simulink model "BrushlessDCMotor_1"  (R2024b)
settings: Solver=ode4  StartTime=0  StopTime=3  FixedStep=Ts  MaxStep=1e-6  RelTol=1e-6  AbsTol=1e-6  EnableMultiTasking=on
PreLoadFcn:
  | assignin('base','Ts',[5e-6])
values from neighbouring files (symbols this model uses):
  A = [-Rs/Ls,  -Ke/Ls    [dc_motor_hinf.m]
  B = 0.001    [dc_motor_hinf.m]
  J = 0.0008    [dc_motor_hinf.m]
  Ke = 0.175    [dc_motor_hinf.m]
  Kt = 0.175    [dc_motor_hinf.m]
  Ls = 8.5e-3    (= 0.0085)    [dc_motor_hinf.m]
  Rs = 2.875    [dc_motor_hinf.m]
  Ts = 5e-6    (= 5e-06)    [dc_motor_hinf.m]
undefined symbols (not defined in the file or in its folder): axis, behind, by, degrees, den_cl, established, Flux, linkage, magnets, modified, num_cl, Park, phase, V
libraries: simulink x6, spsVoltageMeasurementLib x2, spsControlledVoltageSourceLib x1, cstblocks x1, spsPermanentMagnetSynchronousMachineLib x1, spsThreePhaseSeriesRLCLoadLib x1, spsUniversalBridgeLib x1, spspowerguiLib x1

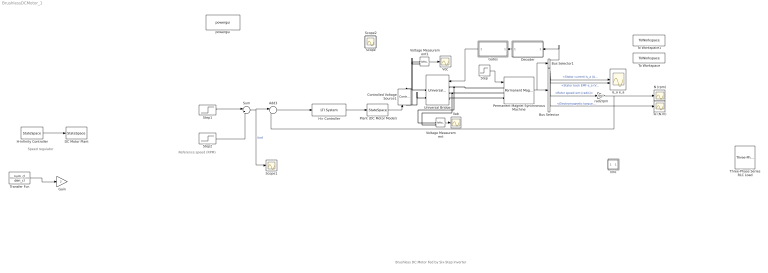
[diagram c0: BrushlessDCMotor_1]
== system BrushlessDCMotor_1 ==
  note: Brushless DC Motor Fed by Six-Step Inverter
  note: Speed regulator
  note: Reference speed (RPM)
  Add3 : Sum  Inputs=|+-
  Bus Selector : BusSelector  OutputSignals=Stator current is_a (A),Stator back EMF e_a (V),Rotor speed wm (rad/s),Electromagnetic torque Te (N*m)
  Bus Selector1 : BusSelector  OutputSignals=Hall effect signal h_a,Hall effect signal h_b,Hall effect signal h_c  OutputAsBus=on
  Controlled Voltage Source1 : spsControlledVoltageSourceLib/Controlled Voltage Source  Initialize=on  Source_Type=AC  Amplitude=500  Phase=0  Frequency=50  Measurements=None
  DC Motor Plant : StateSpace  Commented=on  A=[-Rs/Ls, -Ke/Ls; Kt/J, -B/J]  B=[1/Ls; 0]  C=[0, 1]  InitialCondition=0  ContinuousStateAttributes=''sys'
  Decoder : Subsystem
  Gain : Gain  Commented=on  Gain=2
  Gates : Subsystem
  H-Infinity Controller : StateSpace  Commented=on  InitialCondition=0  ContinuousStateAttributes=''K'
  H∞ Controller : cstblocks/LTI System  sys=K_discrete  IC=[]  PadeOrder=0
  Info : Subsystem
  N (rpm) : Scope
  Permanent Magnet Synchronous Machine : spsPermanentMagnetSynchronousMachineLib/Permanent Magnet Synchronous Machine  NbPhases=3  FluxDistribution=Trapezoidal  RotorType=Round  MechanicalLoad=Torque Tm  PresetModel=No  ShowDetailedParameters=on  MeasurementBus=off  Resistance=2.8750  Inductance=8.5e-3  dqInductances=[8.5e-3, 8.5e-3]  La=0.000835  MachineConstant=Flux linkage established by magnets (V.s)  Flux=0.175  VoltageCst=146.6077  TorqueCst=1.4  Flat=120  Mechanical=[ 0.8e-3, 1e-3 4]  PolePairs=4  InitialConditions=[0,0, 0,0]  InitialConditions5ph=[0 0 0 0 0 0]  RefAngle=90 degrees behind phase A axis (modified Park)  IterativeDiscreteModel=Trapezoidal non iterative  TsBlock=-1  TsPowergui=0
  Plant (DC Motor Model) : StateSpace  A=|  B=|  C=[0, 1]  D=0  InitialCondition=0
      | [-338.2353, -20.5882;
      |  218.75, -1.25]
      | [117.6471;
      |  0]
  Scope1 : Scope
  Step : Step  Time=.1  After=0  SampleTime=0
  Step1 : Step  Time=1.3  Before=3000  After=2500  SampleTime=0
  Step2 : Step  Time=2.5  After=500  SampleTime=0
  Sum : Sum  Inputs=|++
  Te (N.m) : Scope
  Three-Phase Series RLC Load : spsThreePhaseSeriesRLCLoadLib/Three-Phase Series RLC Load  LConnTagsString=A|B|C  Configuration=Y (grounded)  NominalVoltage=400  Vabc=[1e3 1e3 1e3]  Vabcp=[1e3 1e3 1e3]  NominalFrequency=50  UnbalancedPower=off  ActivePower=10e3  InductivePower=200  CapacitivePower=0  Pabc=[10e3 9e3 11e3]  QLabc=[100 90 110]  QCabc=[100 90 110]  Pabcp=[10e3 9e3 11e3]  QLabcp=[100 90 110]  QCabcp=[100 90 110]  Measurements=None  LoadType=constant Z
  To Workspace : ToWorkspace  VariableName=y_data  SaveFormat=Timeseries  SampleTime=-1
  To Workspace1 : ToWorkspace  VariableName=u_data  SaveFormat=Timeseries  SampleTime=-1
  Transfer Fcn : TransferFcn  Commented=on  Numerator=num_cl  Denominator=den_cl
  Universal Bridge : spsUniversalBridgeLib/Universal Bridge  Arms=3  SnubberResistance=10000  SnubberCapacitance=1e-6  Device=MOSFET / Diodes  Ron=1e-3  Lon=0  ForwardVoltages="[  0  0  ]"  ForwardVoltage=0  GTOparameters=[ 10e-6 , 20e-6 ]  IGBTparameters=[ 1e-6 , 2e-6 ]  Measurements=None  Measurements_2=None  converterType=Rectifier
  Vab : Scope
  Vdc : Scope
  Voltage Measurement : spsVoltageMeasurementLib/Voltage Measurement  PhasorSimulation=off  OutputType=Complex  PSBequivalent=0
  Voltage Measurement1 : spsVoltageMeasurementLib/Voltage Measurement  PhasorSimulation=off  OutputType=Complex  PSBequivalent=0
  is_a e_a : Scope  NumInputPorts=2
  powergui : spspowerguiLib/powergui  Priority=2  SimulationMode=Discrete  SampleTime=Ts  frequency=60  Iterations=50  frequencyindice=0  Pbase=100e6  ErrMax=1e-4  UnitsV=kV  UnitsW=MW  buscounter=0  FunctionMessages=off  echomessages=off  EnableUseOfTLC=off  CurrentSourceSwitches=off  DisableSnubberDevices=off  DisableRonSwitches=off  DisableVfSwitches=off  DisplayEquations=off  AutomaticDiscreteSolvers=off  SolverType=Tustin/Backward Euler (TBE)  Interpol=off  ExternalGateDelay=off  methode=off  Ts=0  x0status=blocks  SPID=off  SwTol=0  HookPort=off  NonlinearTolerance=1e-4  nMaxIteration=100  ContinueOnMaxIteration=off  RestoreLinks=warning  ResistiveCurrentMeasurement=off  Frange=[0:2:500]  Ylog=off  Xlog=on  ShowGrid=off  save=off  variable=ZData  structure=0  ZoomFFT=on  StartTime=0.0  cycles=1  DisplayStyle=1  fundamental=60  FreqAxis=off  MaxFrequency=1000  frequencyindicesteady=1  RmsSteady=1  display=off
  rad2rpm : Gain  Gain=30/pi
  Scope : Scope
  Scope2 : Scope
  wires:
  Step/1 -> Permanent Magnet Synchronous Machine/1
  Add3/1 -> H∞ Controller/1
  Gates/1(Gates) -> Universal Bridge/1
  Decoder/1(emf_abc) -> Gates/1("emf_abc ")
  rad2rpm/1 -> N (rpm)/1, Add3/2
  Voltage Measurement/1 -> Vab/1
  Voltage Measurement1/1 -> Vdc/1
  Bus Selector/1 -> is_a e_a/1  "<Stator current is_a (A)>"
  Permanent Magnet Synchronous Machine/1 -> Bus Selector/1, Bus Selector1/1
  Bus Selector1/1 -> Decoder/1("Hall ")
  Bus Selector/2 -> is_a e_a/2  "<Stator back EMF e_a (V)>"
  Bus Selector/3 -> rad2rpm/1  "<Rotor speed wm (rad/s)>"
  Bus Selector/4 -> Te (N.m)/1  "<Electromagnetic torque Te (N*m)>"
  Transfer Fcn/1 -> Gain/1
  Sum/1 -> Scope1/1, Add3/1  "Vref"
  Step2/1 -> Sum/2
  Step1/1 -> Sum/1
  DC Motor Plant/1 -> ?
  H-Infinity Controller/1 -> DC Motor Plant/1
  Gain/1 -> ?
  H∞ Controller/1 -> Plant (DC Motor Model)/1
  Plant (DC Motor Model)/1 -> Controlled Voltage Source1/1
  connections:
  Universal Bridge/LConn1 -- Permanent Magnet Synchronous Machine/LConn1 -- Voltage Measurement/LConn1
  Universal Bridge/LConn2 -- Permanent Magnet Synchronous Machine/LConn2 -- Voltage Measurement/LConn2
  Controlled Voltage Source1/RConn1 -- Universal Bridge/RConn1 -- Voltage Measurement1/LConn1
  Controlled Voltage Source1/LConn1 -- Universal Bridge/RConn2 -- Voltage Measurement1/LConn2
  Universal Bridge/LConn3 -- Permanent Magnet Synchronous Machine/LConn3

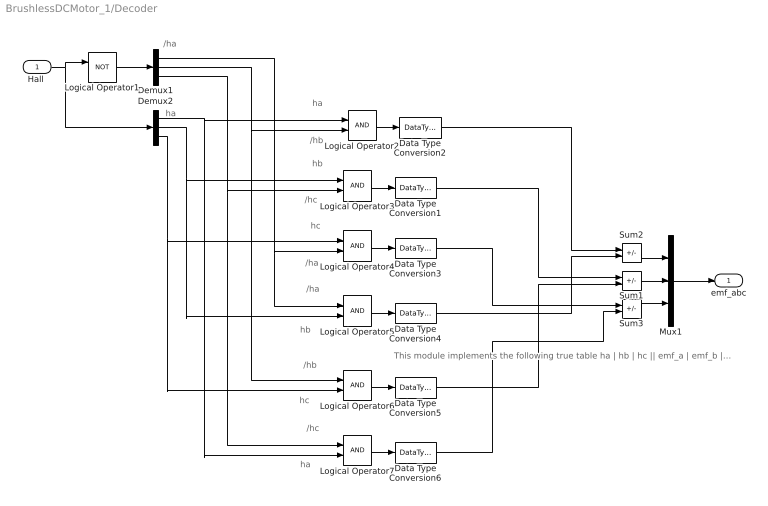
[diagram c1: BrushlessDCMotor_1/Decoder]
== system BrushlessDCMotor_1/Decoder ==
  note: /ha
  note: ha
  note: ha
  note: /hb
  note: hb
  note: /hc
  note: hc
  note: /ha
  note: /ha
  note: hb
  note: /hb
  note: hc
  note: /hc
  note: ha
  note: This module implements the following true table ha | hb | hc || emf_a | emf_b | emf_c -------------------------------------------------------------------------------- 0 0 0 0 0 0 0 0 1 0 -1 +1 0 1 0 -1 +1 0 0 1 1 -1 0 +1 1 0 0 +1 0 -1 1 0 1 +1 -1 0 1 1 0 0 +1 -1 1 1 1 0 0 0
  "Hall " : Inport
  Data Type Conversion{1..6} (6 alike) : DataTypeConversion
  Demux1 : Demux  Outputs=3
  Demux2 : Demux  Outputs=3
  Logical Operator1 : Logic  Operator=NOT  AllPortsSameDT=off  OutDataTypeStr=boolean
  Logical Operator{2..7} (6 alike) : Logic  AllPortsSameDT=off  OutDataTypeStr=boolean
  Mux1 : Mux  Inputs=3
  Sum1 : Sum  Inputs=+-  OutDataTypeStr=double
  Sum2 : Sum  Inputs=+-  OutDataTypeStr=double
  Sum3 : Sum  Inputs=+-  OutDataTypeStr=double
  emf_abc : Outport  VectorParamsAs1DForOutWhenUnconnected=off
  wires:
  "Hall "/1 -> Logical Operator1/1, Demux2/1
  Logical Operator1/1 -> Demux1/1
  Demux2/3 -> Logical Operator4/1, Logical Operator6/2
  Demux2/2 -> Logical Operator3/1, Logical Operator5/2
  Demux2/1 -> Logical Operator2/1, Logical Operator7/2
  Demux1/3 -> Logical Operator3/2, Logical Operator7/1
  Demux1/2 -> Logical Operator2/2, Logical Operator6/1
  Demux1/1 -> Logical Operator4/2, Logical Operator5/1
  Logical Operator2/1 -> Data Type Conversion2/1
  Sum2/1 -> Mux1/1
  Sum1/1 -> Mux1/2
  Sum3/1 -> Mux1/3
  Mux1/1 -> emf_abc/1
  Logical Operator3/1 -> Data Type Conversion1/1
  Logical Operator4/1 -> Data Type Conversion3/1
  Logical Operator5/1 -> Data Type Conversion4/1
  Logical Operator6/1 -> Data Type Conversion5/1
  Logical Operator7/1 -> Data Type Conversion6/1
  Data Type Conversion2/1 -> Sum2/1
  Data Type Conversion4/1 -> Sum2/2
  Data Type Conversion1/1 -> Sum1/1
  Data Type Conversion5/1 -> Sum1/2
  Data Type Conversion3/1 -> Sum3/1
  Data Type Conversion6/1 -> Sum3/2

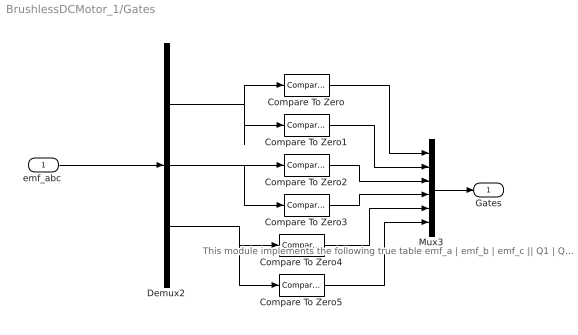
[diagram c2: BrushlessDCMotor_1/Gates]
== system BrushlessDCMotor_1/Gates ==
  note: This module implements the following true table emf_a | emf_b | emf_c || Q1 | Q2 | Q3 | Q4 | Q5 | Q6 ------------------------------------------------------------------------------------------------------------------ 0 0 0 0 0 0 0 0 0 0 -1 +1 0 0 0 1 1 0 -1 +1 0 0 1 1 0 0 0 -1 0 +1 0 1 0 0 1 0 +1 0 -1 1 0 0 0 0 1 +1 -1 0 1 0 0 1 0 0 0 +1 -1 0 0 1 0 0 1 0 0 0 0 0 0 0 0 0
  "emf_abc " : Inport
  Compare To Zero : simulink/Logic and Bit Operations/Compare To Zero  relop=>  OutDataTypeStr=boolean  ZeroCross=off
  Compare To Zero1 : simulink/Logic and Bit Operations/Compare To Zero  relop=<  OutDataTypeStr=boolean  ZeroCross=off
  Compare To Zero2 : simulink/Logic and Bit Operations/Compare To Zero  relop=>  OutDataTypeStr=boolean  ZeroCross=off
  Compare To Zero3 : simulink/Logic and Bit Operations/Compare To Zero  relop=<  OutDataTypeStr=boolean  ZeroCross=off
  Compare To Zero4 : simulink/Logic and Bit Operations/Compare To Zero  relop=>  OutDataTypeStr=boolean  ZeroCross=off
  Compare To Zero5 : simulink/Logic and Bit Operations/Compare To Zero  relop=<  OutDataTypeStr=boolean  ZeroCross=off
  Demux2 : Demux  Outputs=3
  Mux3 : Mux  Inputs=6
  Gates : Outport  VectorParamsAs1DForOutWhenUnconnected=off
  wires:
  "emf_abc "/1 -> Demux2/1
  Mux3/1 -> Gates/1
  Demux2/1 -> Compare To Zero/1, Compare To Zero1/1
  Demux2/2 -> Compare To Zero2/1, Compare To Zero3/1
  Demux2/3 -> Compare To Zero4/1, Compare To Zero5/1
  Compare To Zero/1 -> Mux3/1
  Compare To Zero1/1 -> Mux3/2
  Compare To Zero2/1 -> Mux3/3
  Compare To Zero3/1 -> Mux3/4
  Compare To Zero4/1 -> Mux3/5
  Compare To Zero5/1 -> Mux3/6

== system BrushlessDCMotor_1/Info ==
